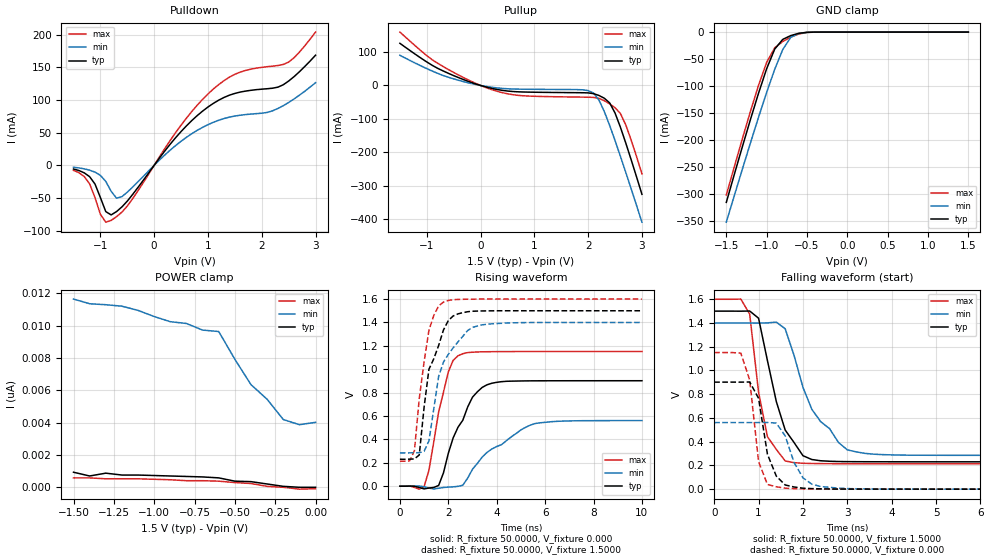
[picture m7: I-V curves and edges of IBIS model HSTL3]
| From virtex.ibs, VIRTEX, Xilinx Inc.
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|   Model HSTL3
[Model]   HSTL3
Model_type   I/O
Polarity   Non-Inverting
Enable   Active-Low
Vinl =   0.800V
Vinh =   1.000V
Vmeas =   0.9000V
Cref =  20.0000pF
Rref =  50.0000
Vref =   1.5000V
C_comp   6.5000pF   5.0000pF   8.0000pF
[Temperature Range]   27.0000   100.0000   0.000
[Voltage Range]   1.5000V   1.4000V   1.6000V
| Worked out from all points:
|   slope of the pulldown table from 0 to 0.225 V, typ, clamps not added: 9.08 ohm
|   slope of the pullup table from 0 to 0.225 V, typ, clamps not added: 24.4 ohm
|   GND clamp passes 1 mA (typ) near -0.53 V on its own axis
|   rising waveform, R_fixture 50.0000, V_fixture 0.000: 20-80 % time 1.03ns typ, 1.88ns min, 658ps max; typ from 0 V to 0.901 V
|   rising waveform, R_fixture 50.0000, V_fixture 1.5000: 20-80 % time 759ps typ, 889ps min, 508ps max; typ from 0.23 V to 1.5 V
|   falling waveform, R_fixture 50.0000, V_fixture 1.5000: 20-80 % time 517ps typ, 848ps min, 328ps max; typ from 1.5 V to 0.23 V
|   falling waveform, R_fixture 50.0000, V_fixture 0.000: 20-80 % time 305ps typ, 374ps min, 203ps max; typ from 0.902 V to 0 V
[Pulldown]
| voltage   I(typ)   I(min)   I(max)
-1.5V     -5.7mA     -3mA       -7.8mA
-1.2V     -17.5mA    -7.5mA     -28.5mA
-1V       -49.46mA   -15.4mA    -75.13mA
-900mV    -71mA      -24.74mA   -87.2mA
-800mV    -76.04mA   -39.84mA   -84.48mA
-600mV    -63.8mA    -48.08mA   -71.74mA
400mV     42.41mA    30.33mA    50.21mA
1.1V      94.87mA    65.89mA    116.9mA
1.6V      112.2mA    76.72mA    142.8mA
2.1V      117.3mA    80.97mA    151.1mA
2.5V      129.1mA    96.26mA    158.1mA
3V        168.7mA    126.5mA    204.1mA
[Pullup]
| voltage   I(typ)   I(min)   I(max)
-1.5V     125.9mA    90.12mA    159.4mA
-800mV    51.38mA    36.35mA    66.49mA
200mV     -8.409mA   -5.19mA    -12mA
800mV     -19.49mA   -11.15mA   -30.84mA
1.9V      -21.68mA   -12.97mA   -34.78mA
2.1V      -24.39mA   -22.73mA   -35.61mA
2.2V      -29.81mA   -43.31mA   -38.52mA
2.4V      -52.01mA   -119.4mA   -54.99mA
2.5V      -82.26mA   -164.5mA   -66.45mA
2.6V      -124.7mA   -211.5mA   -83.78mA
2.7V      -172.1mA   -259.7mA   -118mA
3V        -325mA     -408.2mA   -263.8mA
[GND_clamp]
| voltage   I(typ)   I(min)   I(max)
-1.5V     -315.9mA   -352.6mA   -302.3mA
-1.3V     -212.2mA   -253.8mA   -197.4mA
-1.2V     -161.8mA   -205.3mA   -146.7mA
-1.1V     -113.2mA   -157.8mA   -98.56mA
-1V       -68.04mA   -112mA     -56.27mA
-900mV    -31.6mA    -69.09mA   -29.2mA
-800mV    -13.5mA    -32.34mA   -17.42mA
-700mV    -6.408mA   -9.455mA   -9.303mA
-600mV    -2.237mA   -2.349mA   -3.538mA
-500mV    -423.5uA   -545.3uA   -698.2uA
-400mV    -42.44uA   -91.25uA   -59.93uA
1.5V      0A         3.871nA    -232.8pA
[POWER_clamp]
| voltage   I(typ)   I(min)   I(max)
-1.5V     931.3pA    11.64nA    582.1pA
-1.4V     698.5pA    11.35nA    582.1pA
-1.3V     873.1pA    11.29nA    523.9pA
-1.2V     756.7pA    11.2nA     523.9pA
-900mV    698.5pA    10.24nA    465.7pA
-700mV    640.3pA    9.721nA    407.5pA
-600mV    582.1pA    9.633nA    378.3pA
-400mV    349.2pA    6.345nA    232.8pA
-300mV    203.7pA    5.442nA    58.21pA
-200mV    58.21pA    4.191nA    0A
-100mV    0A         3.871nA    -116.4pA
0V        0A         4.016nA    -87.31pA
[Ramp]
| variable   typ   min   max
dV/dt_r   0.5408/1.0679n   0.3365/1.8265n   0.6906/0.6208n
dV/dt_f   0.7618/0.4372n   0.6689/0.8417n   0.8318/0.3121n
R_load = 50.0000
[Rising Waveform]
R_fixture = 50.0000
V_fixture = 0.000
| time   V(typ)   V(min)   V(max)
0s        0V         0V         0V
1ns       -22.84mV   -4.376mV   -3.153mV
1.2ns     -15.39mV   -15.88mV   136.3mV
1.6ns     6.461mV    -16.9mV    633.8mV
2ns       281.1mV    -7.623mV   977mV
2.4ns     503.9mV    -1.114mV   1.115V
3ns       761.1mV    145.4mV    1.145V
3.8ns     879.9mV    318.3mV    1.149V
5.6ns     900.6mV    536.4mV    1.151V
10ns      901.3mV    560.9mV    1.151V
[Rising Waveform]
R_fixture = 50.0000
V_fixture = 1.5000
V_fixture_min = 1.4000
V_fixture_max = 1.6000
| time   V(typ)   V(min)   V(max)
0s        230.3mV    284.9mV    213.5mV
400ps     231.3mV    285.1mV    216.3mV
600ps     233.3mV    285.9mV    303.6mV
800ps     267.2mV    286.4mV    748.7mV
1.2ns     999.6mV    387.1mV    1.333V
1.6ns     1.202V     938.2mV    1.54V
1.8ns     1.335V     1.06V      1.573V
2.2ns     1.454V     1.183V     1.593V
3.4ns     1.498V     1.379V     1.599V
10ns      1.499V     1.399V     1.599V
[Falling Waveform]
R_fixture = 50.0000
V_fixture = 1.5000
V_fixture_min = 1.4000
V_fixture_max = 1.6000
| time   V(typ)   V(min)   V(max)
0s        1.5V       1.4V       1.6V
600ps     1.5V       1.4V       1.602V
800ps     1.501V     1.4V       1.475V
1ns       1.44V      1.399V     816.4mV
1.2ns     1.083V     1.401V     442.4mV
1.4ns     738.2mV    1.407V     334.8mV
1.6ns     498mV      1.351V     237.9mV
2.2ns     249.9mV    673mV      216.4mV
3ns       232mV      331.1mV    214.3mV
10ns      230.4mV    285.1mV    213.6mV
[Falling Waveform]
R_fixture = 50.0000
V_fixture = 0.000
| time   V(typ)   V(min)   V(max)
0s        901.7mV    561.2mV    1.151V
600ps     901.8mV    561.3mV    1.146V
800ps     903.1mV    561.3mV    919.7mV
1ns       765.6mV    561.3mV    232mV
1.2ns     294.3mV    562mV      39.25mV
1.4ns     109.9mV    556.8mV    20.52mV
1.6ns     35.55mV    449.3mV    8.203mV
2ns       8.481mV    95.92mV    2.753mV
2.4ns     2.878mV    22.21mV    1.252mV
10ns      101.2uV    121.3uV    94.98uV
